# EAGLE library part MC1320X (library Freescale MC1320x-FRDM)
Freescale MC1320x RF Daughter Board Connector
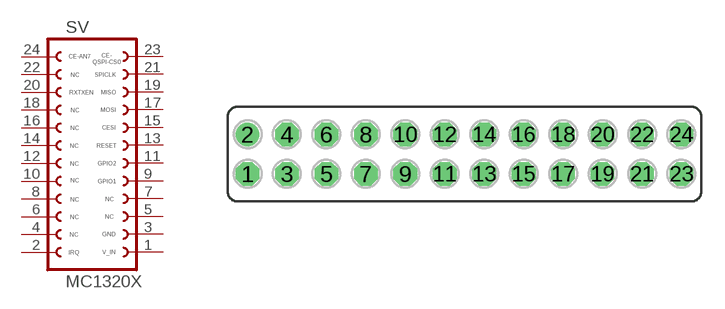
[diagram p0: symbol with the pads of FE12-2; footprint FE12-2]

Designator prefix SV

## MC1320X  [FE12-2]
1  1  pas
2  2  pas
3  3  pas
4  4  pas
5  5  pas
6  6  pas
7  7  pas
8  8  pas
9  9  pas
10  10  pas
11  11  pas
12  12  pas
13  13  pas
14  14  pas
15  15  pas
16  16  pas
17  17  pas
18  18  pas
19  19  pas
20  20  pas
21  21  pas
22  22  pas
23  23  pas
24  24  pas

## Footprint FE12-2 (pad centres in mm)
Female Pin Header for Freescale MC1320x RF Daughter Card
drill 1.016 octagon: 1 -13.97,-1.27; 3 -11.43,-1.27; 4 -11.43,1.27; 5 -8.89,-1.27; 6 -8.89,1.27; 7 -6.35,-1.27; 8 -6.35,1.27; 9 -3.81,-1.27; 10 -3.81,1.27; 11 -1.27,-1.27; 12 -1.27,1.27; 13 1.27,-1.27; 14 1.27,1.27; 15 3.81,-1.27; 16 3.81,1.27; 17 6.35,-1.27; 18 6.35,1.27; 19 8.89,-1.27; 20 8.89,1.27; 21 11.43,-1.27; 22 11.43,1.27; 23 13.97,-1.27; 24 13.97,1.27
drill 1.016: 2 -13.97,1.27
